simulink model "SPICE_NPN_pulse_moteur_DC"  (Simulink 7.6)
settings: Solver=ode15s  StartTime=0.0  StopTime=1  RelTol=1e-3
StopFcn:
  | close all, clc
  | load pos_vit.mat
  | plotyy(x(1,:),x(2,:),x(1,:),x(3,:))
  | title('vitesse et position angulaires')
  | grid
  | 
  | figure
  | plotyy(x(1,:),x(5,:),x(1,:),x(6,:))
  | title('Courant de base et d''émetteur du transistor')
  | xlabel('temps')
  | grid
  | 
  | delete pos_vit.mat
libraries: fl_lib x9, nesl_utility x6, elec_lib x5

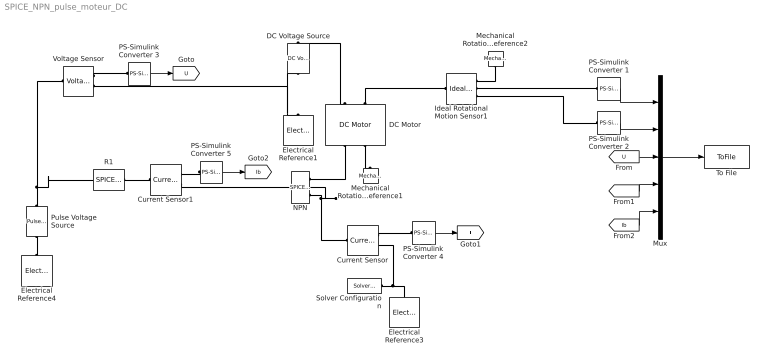
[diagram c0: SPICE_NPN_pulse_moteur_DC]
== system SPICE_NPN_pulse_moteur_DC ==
  Current Sensor : fl_lib/Electrical/Electrical Sensors/Current Sensor  DialogController=NetworkEngine.DynNeDlgSource  SystemSampleTime=-1  i1_Log=off  v1_Log=off  LocalVarNames=|i1|v1  LocalVarDescs=|i1|v1  LocalVarLogging=[0 0]
  Current Sensor1 : fl_lib/Electrical/Electrical Sensors/Current Sensor  DialogController=NetworkEngine.DynNeDlgSource  SystemSampleTime=-1  i1_Log=off  v1_Log=off  LocalVarNames=|i1|v1  LocalVarDescs=|i1|v1  LocalVarLogging=[0 0]
  DC Motor : elec_lib/Actuators & Drivers/Rotational Actuators/DC Motor  DialogController=NetworkEngine.DynNeDlgSource  SystemSampleTime=-1  parameterization=1  Ra=3.9 Ohm  La=1.2e-05 H  emf_or_torque=1  Kv=7.2e-05 V/rpm  Ki=6.876e-04 N*m/A  T_stall=2.4e-04 N*m  w_max=1.91e+04 rpm  w_rated=1.5e+04 rpm  P_rated=0.08 W  V_rated=1.5 V  J=0.01 g*cm^2  lam=1e-08 N*m/(rad/s)  speed0=0 rpm  current_Log=off  voltage_Log=off  power_Log=off  i2r_Log=off  torque_Log=off  speed_Log=off  LocalVarNames=|current|voltage|power|i2r|torque|speed  LocalVarDescs=|Current (A)|Voltage (V)|Power (W)|Electrical losses (W)|Torque (Nm)|Angular speed (rad/s)  LocalVarLogging=[0 0 0 0 0 0]
  DC Voltage Source : elec_lib/Additional Components/SPICE-Compatible Components/Sources/DC Voltage Source  DialogController=NetworkEngine.DynNeDlgSource  SystemSampleTime=-1  DC=12 V  current_Log=off  voltage_Log=off  power_Log=off  LocalVarNames=|current|voltage|power  LocalVarDescs=|Current (A)|Voltage (V)|Power (W)  LocalVarLogging=[0 0 0]
  Electrical Reference1 : fl_lib/Electrical/Electrical Elements/Electrical Reference  DialogController=NetworkEngine.DynNeDlgSource  SystemSampleTime=-1  i_Log=off  LocalVarNames=|i  LocalVarDescs=|i  LocalVarLogging=0
  Electrical Reference3 : fl_lib/Electrical/Electrical Elements/Electrical Reference  DialogController=NetworkEngine.DynNeDlgSource  SystemSampleTime=-1  i_Log=off  LocalVarNames=|i  LocalVarDescs=|i  LocalVarLogging=0
  Electrical Reference4 : fl_lib/Electrical/Electrical Elements/Electrical Reference  DialogController=NetworkEngine.DynNeDlgSource  SystemSampleTime=-1  i_Log=off  LocalVarNames=|i  LocalVarDescs=|i  LocalVarLogging=0
  Ideal Rotational Motion Sensor1 : fl_lib/Mechanical/Mechanical Sensors/Ideal Rotational Motion Sensor  DialogController=NetworkEngine.DynNeDlgSource  SystemSampleTime=-1  offset=0 rad  w_Log=off  t_Log=off  phi_Log=off  LocalVarNames=|w|t|phi  LocalVarDescs=|w|t|phi  LocalVarLogging=[]
  Mechanical Rotational Reference1 : fl_lib/Mechanical/Rotational Elements/Mechanical Rotational Reference  DialogController=NetworkEngine.DynNeDlgSource  SystemSampleTime=-1  t_Log=off  LocalVarNames=|t  LocalVarDescs=|t  LocalVarLogging=[]
  Mechanical Rotational Reference2 : fl_lib/Mechanical/Rotational Elements/Mechanical Rotational Reference  DialogController=NetworkEngine.DynNeDlgSource  SystemSampleTime=-1  t_Log=off  LocalVarNames=|t  LocalVarDescs=|t  LocalVarLogging=[]
  Mux : Mux  Inputs=5
  NPN : elec_lib/Additional Components/SPICE-Compatible Components/Semiconductor Devices/SPICE NPN  DialogController=NetworkEngine.DynNeDlgSource  SystemSampleTime=-1  AREA=1 cm^2  SCALE=1  IS=1e-16 A/m^2  BF=10  NF=1  VAF=Inf V  IKF=Inf A/m^2  ISE=0 A/m^2  NE=1.5  BR=1  NR=1  VAR=Inf V  IKR=Inf A/m^2  ISC=0 A/m^2  NC=2  RB=0 m^2*Ohm  IRB=Inf A/m^2  RBM=0 m^2*Ohm  RE=0 m^2*Ohm  RC=0 m^2*Ohm  C_param=1  CJE=0 F/m^2  VJE=0.75 V  MJE=0.33  TF=0 s  XTF=0  VTF=Inf V  ITF=0 A/m^2  CJC=0 F/m^2  VJC=0.75 V  MJC=0.33  XCJC=1  TR=0 s  CJS=0 F/m^2  VJS=0.75 V  MJS=0  T_param=1  XTB=0  EG=1.11 eV  XTI=3  FC=0.5  TOFFSET=0 K  TFIXED=300.15 K  TMEAS=300.15 K  IC_given=1  ICVBE=0 V  ICVCE=0 V  LocalVarLogging=[]
  PS-Simulink Converter {1..5} (5 alike) : nesl_utility/PS-Simulink Converter  DialogController=NetworkEngine.DynNeUtilDlgSource  SystemSampleTime=-1  PhysicalDomain=network_engine_domain  LeftPortType=input  RightPortType=output  SubClassName=ps_output  Unit=1  AffineConversion=off
  Pulse Voltage  Source : elec_lib/Additional Components/SPICE-Compatible Components/Sources/Pulse Voltage Source  DialogController=NetworkEngine.DynNeDlgSource  SystemSampleTime=-1  V1=0 V  V2=12 V  TD=0 s  TR=1e-09 s  TF=1e-09 s  PW=5 s  PER=20 s  voltage_Log=off  LocalVarNames=|voltage  LocalVarDescs=|Voltage (V)  LocalVarLogging=0
  R1 : elec_lib/Additional Components/SPICE-Compatible Components/Passive Devices/SPICE Resistor  DialogController=NetworkEngine.DynNeDlgSource  SystemSampleTime=-1  SCALE=1  R_param=1  R=10 kOhm  RSH=0 Ohm  LENGTH=1e-06 m  WIDTH=1e-06 m  NARROW=0 m  T_param=1  TC1=0 1/K  TC2=0 1/K^2  TOFFSET=0 K  TFIXED=300.15 K  TMEAS=300.15 K  LocalVarLogging=[]
  Solver Configuration : nesl_utility/Solver Configuration  DialogController=NetworkEngine.DynNeUtilDlgSource  SystemSampleTime=-1  PhysicalDomain=network_engine_domain  LeftPortType=input  RightPortType=generic  SubClassName=solver  Accelerate=off  Profile=off  ResidualTolerance=1e-9  MaxNonlinIter=12  MaxModeIter=2  DoFixedCost=off  UseLocalSampling=off  DoDC=off  LinearAlgebra=Sparse  LocalSolverSampleTime=.001  LocalSolverChoice=NE_BACKWARD_EULER_ADVANCER  UseLocalSolver=off
  To File : ToFile  Filename=pos_vit.mat  MatrixName=x
  Voltage Sensor : fl_lib/Electrical/Electrical Sensors/Voltage Sensor  DialogController=NetworkEngine.DynNeDlgSource  SystemSampleTime=-1  i1_Log=off  v1_Log=off  LocalVarNames=|i1|v1  LocalVarDescs=|i1|v1  LocalVarLogging=[0 0]
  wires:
  PS-Simulink Converter 1/1 -> Mux/1
  Mux/1 -> To File/1
  PS-Simulink Converter 2/1 -> Mux/2
  PS-Simulink Converter 3/1 -> [U]
  [U] -> Mux/3
  [I] -> Mux/4
  PS-Simulink Converter 4/1 -> [I]
  PS-Simulink Converter 5/1 -> [Ib]
  [Ib] -> Mux/5
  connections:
  DC Motor/RConn1 -- NPN/RConn1
  NPN/RConn3 -- NPN/RConn2 -- Current Sensor/LConn1
  Voltage Sensor/RConn2 -- DC Voltage Source/RConn1 -- Electrical Reference1/LConn1
  Current Sensor1/RConn2 -- NPN/LConn1
  DC Voltage Source/LConn1 -- DC Motor/LConn1
  Pulse Voltage  Source/LConn1 -- Voltage Sensor/LConn1 -- R1/RConn1
  Electrical Reference4/LConn1 -- Pulse Voltage  Source/RConn1
  Mechanical Rotational Reference2/LConn1 -- Ideal Rotational Motion Sensor1/RConn1
  Ideal Rotational Motion Sensor1/RConn2 -- PS-Simulink Converter 1/LConn1
  Ideal Rotational Motion Sensor1/RConn3 -- PS-Simulink Converter 2/LConn1
  Voltage Sensor/RConn1 -- PS-Simulink Converter 3/LConn1
  Solver Configuration/RConn1 -- Electrical Reference3/LConn1 -- Current Sensor/RConn2
  Current Sensor/RConn1 -- PS-Simulink Converter 4/LConn1
  DC Motor/LConn2 -- Ideal Rotational Motion Sensor1/LConn1
  DC Motor/RConn2 -- Mechanical Rotational Reference1/LConn1
  R1/LConn1 -- Current Sensor1/LConn1
  PS-Simulink Converter 5/LConn1 -- Current Sensor1/RConn1
